| IBIS file bga144.ibs generated by Viper version: 2021.04.12
[IBIS Ver]   5.0
[Comment Char]   |_char
[File Name]   imxrt1180_c0_bga144_consmr.ibs
[File Rev]   1
[Date]   Mon Sep 20 18:29:30 2021
[Source]   NXP Viper 2021.04.12
[Notes]
[Disclaimer] IMPORTANT NOTICE
  This information is provided on an AS IS basis and without warranty.
  IN NO EVENT SHALL NXP BE LIABLE FOR INCIDENTAL OR CONSEQUENTIAL
  DAMAGES ARISING FROM USE OF THIS INFORMATION. THIS DISCLAIMER OF
  WARRANTY EXTENDS TO THE USER OF THE INFORMATION, AND TO THEIR CUSTOMERS
  OR USERS OF PRODUCTS  AND IS IN LIEU OF ALL WARRANTIES WHETHER EXPRESS,
  IMPLIED, OR STATUTORY, INCLUDING IMPLIED WARRANTIES OF MERCHANTABILITY
  OR FITNESS FOR PARTICULAR PURPOSE.
  NXP does not represent or warrant that the information furnished
  hereunder is free of infringement of any third party patents,
  copyrights, trade secrets, or other intellectual property rights.
  NXP does not represent or warrant that the information is free of
  defect, or that it meets any particular standard, requirements or need
  of the user of the infomation or their customers.
  NXP reserves the right to change the information in this file
  without notice.
   http://www.nxp.com
[Copyright]   (C) Copyright NXP 2004 - 2021, All Rights Reserved.
|   BGA144
[Component]   imxrt1180_bga144
[Manufacturer]   NXP
[Package]
| variable   typ   min   max
R_pkg   0.16359   0.065919   0.31382
L_pkg   2.744e-09   1.070e-09   5.893e-09
C_pkg   6.965e-13   4.261e-13   1.190e-12
[Pin] signal_name   model_name   R_pin   L_pin   C_pin
A1   VSS   GND   NA   NA   NA
A2   GPIO_EMC_B1_16   STGPIO   0.28718   5.367e-09 7.642e-13
A3   GPIO_EMC_B1_09   STGPIO   0.22622   3.718e-09 5.945e-13
A4   GPIO_AON_26   FSGPIO   0.16362   2.856e-09 5.265e-13
A5   GPIO_AON_25   FSGPIO   0.17256   2.828e-09 5.105e-13
A6   GPIO_AON_23   FSGPIO   0.19583   3.160e-09 4.965e-13
A7   GPIO_AON_22   FSGPIO   0.18824   3.176e-09 4.828e-13
A8   GPIO_AON_10   FSGPIO   0.16692   2.583e-09 9.013e-13
A9   GPIO_AON_12   FSGPIO   0.24101   4.139e-09 1.094e-12
A10   GPIO_AON_15   FSGPIO   0.3027   5.713e-09 1.030e-12
A11   GPIO_AON_08   FSGPIO   0.31382   5.893e-09 9.051e-13
A12   VSS   GND   NA   NA   NA
B1   GPIO_EMC_B1_15   STGPIO   0.25831   4.469e-09 6.261e-13
B2   GPIO_EMC_B1_11   STGPIO   0.26853   4.818e-09 7.636e-13
B3   GPIO_EMC_B1_17   STGPIO   0.21276   3.476e-09 6.391e-13
B4   GPIO_AON_27   FSGPIO   0.15742   2.693e-09 5.007e-13
B5   GPIO_AON_24   FSGPIO   0.18906   2.825e-09 5.199e-13
B6   GPIO_AON_05   FSGPIO   0.10031   1.570e-09 1.003e-12
B7   GPIO_AON_03   FSGPIO   0.108   2.043e-09 4.957e-13
B8   GPIO_AON_09   FSGPIO   0.16506   2.661e-09 8.544e-13
B9   GPIO_AON_11   FSGPIO   0.23045   3.870e-09 1.087e-12
B10   GPIO_AON_14   FSGPIO   0.29632   5.573e-09 1.094e-12
B11   GPIO_AON_13   FSGPIO   0.30615   5.598e-09 1.046e-12
B12   GPIO_SD_B2_06   STGPIO   0.24063   4.504e-09 6.685e-13
C1   GPIO_EMC_B1_10   STGPIO   0.19712   2.698e-09 4.825e-13
C2   GPIO_EMC_B1_28   STGPIO   0.077242  1.186e-09 7.516e-13
C3   GPIO_EMC_B1_29   STGPIO   0.10015   1.487e-09 6.582e-13
C4   GPIO_AON_17   FSGPIO   0.10536   1.478e-09 6.818e-13
C5   GPIO_AON_16   FSGPIO   0.10709   1.790e-09 6.038e-13
C6   GPIO_AON_02   FSGPIO   0.067407  1.118e-09 1.122e-12
C7   GPIO_AON_01   FSGPIO   0.078667  1.324e-09 1.017e-12
C8   VSS   GND   NA   NA   NA
C9   GPIO_AON_00   FSGPIO   0.19384   3.878e-09 1.009e-12
C10   GPIO_SD_B2_07   STGPIO   0.23187   4.557e-09 7.771e-13
C11   GPIO_SD_B2_11   STGPIO   0.21729   3.877e-09 6.591e-13
C12   GPIO_SD_B2_04   STGPIO   0.19371   3.729e-09 6.738e-13
D1   GPIO_EMC_B1_30   STGPIO   0.18787   2.739e-09 4.927e-13
D2   GPIO_EMC_B1_14   STGPIO   0.11531   2.030e-09 7.770e-13
D3   GPIO_EMC_B1_12   STGPIO   0.067604  1.070e-09 7.102e-13
D4   VSS   GND   NA   NA   NA
D5   NVCC_AON   POWER   NA   NA   NA
D6   GPIO_AON_04   FSGPIO   0.10548   1.871e-09 1.190e-12
D7   GPIO_AON_06   FSGPIO   0.16092   3.123e-09 8.741e-13
D8   GPIO_AON_07   FSGPIO   0.22286   4.219e-09 9.805e-13
D9   VSS   GND   NA   NA   NA
D10   GPIO_SD_B2_05   STGPIO   0.11127   1.889e-09 8.982e-13
D11   GPIO_SD_B2_08   STGPIO   0.16622   2.574e-09 7.092e-13
D12   GPIO_SD_B2_09   STGPIO   0.21685   3.842e-09 5.853e-13
E1   GPIO_EMC_B1_32   STGPIO   0.17445   2.614e-09 4.506e-13
E2   GPIO_EMC_B1_31   STGPIO   0.17592   2.545e-09 4.829e-13
E3   GPIO_EMC_B1_13   STGPIO   0.10229   1.568e-09 8.463e-13
E4   GPIO_AON_21   FSGPIO   0.13406   2.508e-09 8.079e-13
E5   GPIO_AON_20   FSGPIO   0.1388   2.497e-09 8.535e-13
E6   GPIO_AON_19   FSGPIO   0.20153   3.516e-09 9.171e-13
E7   GPIO_AON_18   FSGPIO   0.20448   3.843e-09 9.142e-13
E8   VDD_SOC   POWER   NA   NA   NA
E9   NVCC_SD2   POWER   NA   NA   NA
E10   GPIO_SD_B2_03   STGPIO   0.070294  1.124e-09 8.050e-13
E11   GPIO_SD_B2_01   STGPIO   0.085638  1.305e-09 5.966e-13
E12   GPIO_SD_B2_10   STGPIO   0.16784   2.532e-09 4.453e-13
F1   GPIO_EMC_B1_34   STGPIO   0.17221   2.611e-09 4.420e-13
F2   GPIO_EMC_B1_33   STGPIO   0.18078   2.550e-09 6.132e-13
F3   GPIO_EMC_B1_08   STGPIO   0.11325   1.890e-09 6.770e-13
F4   GPIO_EMC_B1_03   STGPIO   0.11114   2.060e-09 6.860e-13
F5   GPIO_EMC_B1_05   STGPIO   0.11095   2.061e-09 6.978e-13
F6   NVCC_EMC1   POWER   NA   NA   NA
F7   VDD_SOC   POWER   NA   NA   NA
F8   VDD_SOC   POWER   NA   NA   NA
F9   NVCC_SD2   POWER   NA   NA   NA
F10   GPIO_SD_B2_00   STGPIO   0.097558  1.525e-09 6.253e-13
F11   GPIO_SD_B2_02   STGPIO   0.18599   2.795e-09 5.999e-13
F12   ADC_VREFH   NC   0.094419  1.817e-09 5.253e-13
G1   GPIO_EMC_B1_35   STGPIO   0.16837   2.429e-09 4.604e-13
G2   GPIO_EMC_B1_36   STGPIO   0.18715   2.520e-09 6.142e-13
G3   GPIO_EMC_B1_27   STGPIO   0.10364   1.742e-09 6.797e-13
G4   GPIO_EMC_B1_01   STGPIO   0.1415   2.634e-09 7.744e-13
G5   GPIO_EMC_B1_00   STGPIO   0.11834   2.223e-09 7.515e-13
G6   NVCC_EMC1   POWER   NA   NA   NA
G7   VDD_SOC   POWER   NA   NA   NA
G8   VDDA_ADC_3P3   POWER   NA   NA   NA
G9   VDDA_ADC_1P8   POWER   NA   NA   NA
G10   DAC_OUT   NC   0.065919  1.083e-09 6.529e-13
G11   GPIO_AD_30   FSGPIO   0.18141   2.885e-09 5.922e-13
G12   GPIO_AD_31   FSGPIO   0.16864   2.516e-09 4.261e-13
H1   GPIO_EMC_B1_37   STGPIO   0.17602   2.411e-09 5.024e-13
H2   GPIO_EMC_B1_39   STGPIO   0.17575   2.631e-09 4.659e-13
H3   GPIO_EMC_B1_38   STGPIO   0.24055   4.225e-09 7.361e-13
H4   GPIO_EMC_B1_04   STGPIO   0.13736   2.608e-09 7.247e-13
H5   GPIO_EMC_B1_02   STGPIO   0.17915   3.250e-09 7.855e-13
H6   NVCC_EMC1   POWER   NA   NA   NA
H7   GPIO_BBSM_05   NC   0.14691   2.786e-09 8.118e-13
H8   GPIO_BBSM_06   NC   0.13478   2.603e-09 7.785e-13
H9   NVCC_GPIO_AD   POWER   NA   NA   NA
H10   GPIO_AD_18   FSGPIO   0.094077  1.562e-09 6.277e-13
H11   GPIO_AD_19   FSGPIO   0.088023  1.670e-09 4.904e-13
H12   GPIO_AD_29   FSGPIO   0.11929   2.340e-09 4.541e-13
J1   GPIO_EMC_B1_26   STGPIO   0.13411   2.554e-09 4.869e-13
J2   GPIO_EMC_B1_40   STGPIO   0.18514   2.596e-09 5.007e-13
J3   GPIO_EMC_B1_41   STGPIO   0.19787   3.056e-09 5.706e-13
J4   VSS   GND   NA   NA   NA
J5   GPIO_EMC_B1_07   STGPIO   0.12796   2.721e-09 7.157e-13
J6   GPIO_EMC_B1_06   STGPIO   0.1392   3.086e-09 8.299e-13
J7   TEST_MODE   NC   0.25213   4.636e-09 7.670e-13
J8   GPIO_BBSM_00   NC   0.25627   4.609e-09 7.670e-13
J9   VSS   GND   NA   NA   NA
J10   VDDA_1P8_IN   POWER   NA   NA   NA
J11   GPIO_AD_14   FSGPIO   0.10297   1.489e-09 8.353e-13
J12   GPIO_AD_15   FSGPIO   0.10216   1.657e-09 6.078e-13
K1   DCDC_SENSE   POWER   0.18582   2.383e-09 4.766e-13
K2   DCDC_PSWITCH   NC   0.18656   2.611e-09 4.898e-13
K3   DCDC_GND   GND   NA   NA   NA
K4   DCDC_IN_Q   POWER   0.088509  1.651e-09 7.551e-13
K5   ONOFF   NC   0.20344   3.359e-09 6.540e-13
K6   GPIO_BBSM_01   NC   0.073539  1.216e-09 6.201e-13
K7   NVCC_BBSM   POWER   NA   NA   NA
K8   VDD_BBSM_ANA   POWER   NA   NA   NA
K9   VDD_AON_ANA   POWER   NA   NA   NA
K10   GPIO_AD_13   FSGPIO   0.085008  1.325e-09 7.009e-13
K11   GPIO_AD_12   FSGPIO   0.22058   3.187e-09 8.131e-13
K12   GPIO_AD_17   FSGPIO   0.22522   3.387e-09 6.835e-13
L1   DCDC_1P8   POWER   0.086379  1.798e-09 7.307e-13
L2   DCDC_LP   POWER   NA   NA   NA
L3   DCDC_GND   GND   NA   NA   NA
L4   DCDC_IN   POWER   NA   NA   NA
L5   PMIC_ON_REQ   NC   0.17119   2.572e-09 5.895e-13
L6   POR_B   NC   0.16787   2.505e-09 5.617e-13
L7   RTC_XTALO   NC   0.10473   1.522e-09 5.551e-13
L8   VDD_AON_IN   POWER   NA   NA   NA
L9   XTALO   NC   0.11074   1.571e-09 5.999e-13
L10   VSS   GND   NA   NA   NA
L11   CLK1_N   NC   0.21895   3.146e-09 7.817e-13
L12   GPIO_AD_16   FSGPIO   0.22382   3.398e-09 7.083e-13
M1   VSS   GND   NA   NA   NA
M2   DCDC_LP   POWER   NA   NA   NA
M3   DCDC_GND   GND   NA   NA   NA
M4   DCDC_IN   POWER   NA   NA   NA
M5   WAKEUP   NC   0.178   2.735e-09 5.291e-13
M6   VDD_BBSM_IN   POWER   NA   NA   NA
M7   RTC_XTALI   NC   0.11374   1.747e-09 5.677e-13
M8   VDD_AON_DIG   POWER   NA   NA   NA
M9   XTALI   NC   0.11181   1.555e-09 6.216e-13
M10   VDDA_1P0   POWER   NA   NA   NA
M11   CLK1_P   NC   0.22364   3.329e-09 7.427e-13
M12   VSS   GND   NA   NA   NA
[Pin Mapping]   pulldown_ref   pullup_ref
A1   VSS   NC
A2   VSS   NVCC_EMC1
A3   VSS   NVCC_EMC1
A4   VSS   NVCC_AON
A5   VSS   NVCC_AON
A6   VSS   NVCC_AON
A7   VSS   NVCC_AON
A8   VSS   NVCC_AON
A9   VSS   NVCC_AON
A10   VSS   NVCC_AON
A11   VSS   NVCC_AON
A12   VSS   NC
B1   VSS   NVCC_EMC1
B2   VSS   NVCC_EMC1
B3   VSS   NVCC_EMC1
B4   VSS   NVCC_AON
B5   VSS   NVCC_AON
B6   VSS   NVCC_AON
B7   VSS   NVCC_AON
B8   VSS   NVCC_AON
B9   VSS   NVCC_AON
B10   VSS   NVCC_AON
B11   VSS   NVCC_AON
B12   VSS   NVCC_SD2
C1   VSS   NVCC_EMC1
C2   VSS   NVCC_EMC1
C3   VSS   NVCC_EMC1
C4   VSS   NVCC_AON
C5   VSS   NVCC_AON
C6   VSS   NVCC_AON
C7   VSS   NVCC_AON
C8   VSS   NC
C9   VSS   NVCC_AON
C10   VSS   NVCC_SD2
C11   VSS   NVCC_SD2
C12   VSS   NVCC_SD2
D1   VSS   NVCC_EMC1
D2   VSS   NVCC_EMC1
D3   VSS   NVCC_EMC1
D4   VSS   NC
D5   NC   NVCC_AON
D6   VSS   NVCC_AON
D7   VSS   NVCC_AON
D8   VSS   NVCC_AON
D9   VSS   NC
D10   VSS   NVCC_SD2
D11   VSS   NVCC_SD2
D12   VSS   NVCC_SD2
E1   VSS   NVCC_EMC1
E2   VSS   NVCC_EMC1
E3   VSS   NVCC_EMC1
E4   VSS   NVCC_AON
E5   VSS   NVCC_AON
E6   VSS   NVCC_AON
E7   VSS   NVCC_AON
E8   NC   VDD_SOC
E9   NC   NVCC_SD2
E10   VSS   NVCC_SD2
E11   VSS   NVCC_SD2
E12   VSS   NVCC_SD2
F1   VSS   NVCC_EMC1
F2   VSS   NVCC_EMC1
F3   VSS   NVCC_EMC1
F4   VSS   NVCC_EMC1
F5   VSS   NVCC_EMC1
F6   NC   NVCC_EMC1
F7   NC   VDD_SOC
F8   NC   VDD_SOC
F9   NC   NVCC_SD2
F10   VSS   NVCC_SD2
F11   VSS   NVCC_SD2
F12   NC   NC
G1   VSS   NVCC_EMC1
G2   VSS   NVCC_EMC1
G3   VSS   NVCC_EMC1
G4   VSS   NVCC_EMC1
G5   VSS   NVCC_EMC1
G6   NC   NVCC_EMC1
G7   NC   VDD_SOC
G8   NC   VDDA_ADC_3P3
G9   NC   VDDA_ADC_1P8
G10   NC   NC
G11   VSS   NVCC_GPIO_AD
G12   VSS   NVCC_GPIO_AD
H1   VSS   NVCC_EMC1
H2   VSS   NVCC_EMC1
H3   VSS   NVCC_EMC1
H4   VSS   NVCC_EMC1
H5   VSS   NVCC_EMC1
H6   NC   NVCC_EMC1
H7   NC   NC
H8   NC   NC
H9   NC   NVCC_GPIO_AD
H10   VSS   NVCC_GPIO_AD
H11   VSS   NVCC_GPIO_AD
H12   VSS   NVCC_GPIO_AD
J1   VSS   NVCC_EMC1
J2   VSS   NVCC_EMC1
J3   VSS   NVCC_EMC1
J4   VSS   NC
J5   VSS   NVCC_EMC1
J6   VSS   NVCC_EMC1
J7   NC   NC
J8   NC   NC
J9   VSS   NC
J10   NC   VDDA_1P8_IN
J11   VSS   NVCC_GPIO_AD
J12   VSS   NVCC_GPIO_AD
K1   NC   DCDC_SENSE
K2   NC   NC
K3   DCDC_GND   NC
K4   NC   DCDC_IN_Q
K5   NC   NC
K6   NC   NC
K7   NC   NVCC_BBSM
K8   NC   VDD_BBSM_ANA
K9   NC   VDD_AON_ANA
K10   VSS   NVCC_GPIO_AD
K11   VSS   NVCC_GPIO_AD
K12   VSS   NVCC_GPIO_AD
L1   NC   DCDC_1P8
L2   NC   DCDC_LP
L3   DCDC_GND   NC
L4   NC   DCDC_IN
L5   NC   NC
L6   NC   NC
L7   NC   NC
L8   NC   VDD_AON_IN
L9   NC   NC
L10   VSS   NC
L11   NC   NC
L12   VSS   NVCC_GPIO_AD
M1   VSS   NC
M2   NC   DCDC_LP
M3   DCDC_GND   NC
M4   NC   DCDC_IN
M5   NC   NC
M6   NC   VDD_BBSM_IN
M7   NC   NC
M8   NC   VDD_AON_DIG
M9   NC   NC
M10   NC   VDDA_1P0
M11   NC   NC
M12   VSS   NC
|*   Model Selector   *
[Model Selector] STGPIO
BDPROGSCARUDQP_SDMMC_3V3SF_00_SD   PSW=0 High Drive, 1V8 SD
BDPROGSCARUDQP_SDMMC_3V3SF_01_SD   PSW=0 Low Drive,  1V8 SD
BDPROGSCARUDQP_SDMMC_3V3SF_00_MMC   PSW=0 High Drive, 1V8 MMC
BDPROGSCARUDQP_SDMMC_3V3SF_01_MMC   PSW=0 Low Drive,  1V8 MMC
BDPROGSCARUDQP_SDMMC_3V3SF_10   PSW=1 High Drive, 3V3 +/- 10%, SD & 3V3 MMC
BDPROGSCARUDQP_SDMMC_3V3SF_11   PSW=1 Low Drive,  3V3 +/- 10%, SD & 3V3 MMC
BDPROGSCARUDQP_SDMMC_3V3SF_10_5pct  PSW=1 High Drive, 3V3 +/- 5%, SD & 3V3 MMC
BDPROGSCARUDQP_SDMMC_3V3SF_11_5pct  PSW=1 Low Drive,  3V3 +/- 5%, SD & 3V3 MMC
BDPROGSCARUDQP_SDMMC_3V3SF_11_2v7   PSW=1 Low Drive,  2V7 SD & 2V7 MMC
BDPROGSCARUDQP_SDMMC_3V3SF_10_2v7   PSW=1 High Drive, 2V7 SD & 2V7 MMC
[Model Selector] FSGPIO
io_crnrobe1dse0sre0   Normal range in cont mode, 5mA drive strength, without slew rate
io_crnrobe1dse0sre1   Normal range in cont mode, 5mA drive strength, with slew rate
io_crnrobe1dse1sre0   Normal range in cont mode, 10mA drive strength, without slew rate
io_crnrobe1dse1sre1   Normal range in cont mode, 10mA drive strength, with slew rate
io_crdrobe1dse0sre0   Derated range in cont mode, 5mA drive strength, without slew rate
io_crdrobe1dse0sre1   Derated range in cont mode, 5mA drive strength, with slew rate
io_crdrobe1dse1sre0   Derated range in cont mode, 10mA drive strength, without slew rate
io_crdrobe1dse1sre1   Derated range in cont mode, 10mA drive strength, with slew rate
io_crdr2obe1dse0sre0   Derated2 range in cont mode, 5mA drive strength, without slew rate
io_crdr2obe1dse0sre1   Derated2 range in cont mode, 5mA drive strength, with slew rate
io_crdr2obe1dse1sre0   Derated2 range in cont mode, 10mA drive strength, without slew rate
io_crdr2obe1dse1sre1   Derated2 range in cont mode, 10mA drive strength, with slew rate
io_hrobe1dse0sre0   high range mode, 5mA drive strength, without slew rate
io_hrobe1dse0sre1   high range mode, 5mA drive strength, with slew rate
io_hrobe1dse1sre0   high range mode, 10mA drive strength, without slew rate
io_hrobe1dse1sre1   high range mode, 10mA drive strength, with slew rate
io_lrobe1dse0sre0   low range mode, 5mA drive strength, without slew rate
io_lrobe1dse0sre1   low range mode, 5mA drive strength, with slew rate
io_lrobe1dse1sre0   low range mode, 10mA drive strength, without slew rate
io_lrobe1dse1sre1   low range mode, 10mA drive strength, with slew rate
io_crnrobe1dse0sre0_5pct   Narrow range in cont mode, 5mA drive strength, without slew rate
io_crnrobe1dse0sre1_5pct   Narrow range in cont mode, 5mA drive strength, with slew rate
io_crnrobe1dse1sre0_5pct   Narrow range in cont mode, 10mA drive strength, without slew rate
io_crnrobe1dse1sre1_5pct   Narrow range in cont mode, 10mA drive strength, with slew rate
io_hrobe1dse0sre0_5pct   Narrow range in high range mode, 5mA drive strength, without slew rate
io_hrobe1dse0sre1_5pct   Narrow range in high range mode, 5mA drive strength, with slew rate
io_hrobe1dse1sre0_5pct   Narrow range in high range mode, 10mA drive strength, without slew rate
io_hrobe1dse1sre1_5pct   Narrow range in high range mode, 10mA drive strength, with slew rate
|End  [Component] imxrt1180_bga144
| Models and submodels in the file (38): BDPROGSCARUDQP_SDMMC_3V3SF_00_MMC (I/O), BDPROGSCARUDQP_SDMMC_3V3SF_00_SD (I/O), BDPROGSCARUDQP_SDMMC_3V3SF_01_MMC (I/O), BDPROGSCARUDQP_SDMMC_3V3SF_01_SD (I/O), BDPROGSCARUDQP_SDMMC_3V3SF_10 (I/O), BDPROGSCARUDQP_SDMMC_3V3SF_11 (I/O), BDPROGSCARUDQP_SDMMC_3V3SF_10_2v7 (I/O), BDPROGSCARUDQP_SDMMC_3V3SF_11_2v7 (I/O), BDPROGSCARUDQP_SDMMC_3V3SF_10_5pct (I/O), BDPROGSCARUDQP_SDMMC_3V3SF_11_5pct (I/O), io_crnrobe1dse0sre0 (I/O), io_crnrobe1dse0sre1 (I/O), io_crnrobe1dse1sre0 (I/O), io_crnrobe1dse1sre1 (I/O), io_crdrobe1dse0sre0 (I/O), io_crdrobe1dse0sre1 (I/O), io_crdrobe1dse1sre0 (I/O), io_crdrobe1dse1sre1 (I/O), io_crdr2obe1dse0sre0 (I/O), io_crdr2obe1dse0sre1 (I/O), io_crdr2obe1dse1sre0 (I/O), io_crdr2obe1dse1sre1 (I/O), io_hrobe1dse0sre0 (I/O), io_hrobe1dse0sre1 (I/O), io_hrobe1dse1sre0 (I/O), io_hrobe1dse1sre1 (I/O), io_lrobe1dse0sre0 (I/O), io_lrobe1dse0sre1 (I/O), io_lrobe1dse1sre0 (I/O), io_lrobe1dse1sre1 (I/O), io_crnrobe1dse0sre0_5pct (I/O), io_crnrobe1dse0sre1_5pct (I/O), io_crnrobe1dse1sre0_5pct (I/O), io_crnrobe1dse1sre1_5pct (I/O), io_hrobe1dse0sre0_5pct (I/O), io_hrobe1dse0sre1_5pct (I/O), io_hrobe1dse1sre0_5pct (I/O), io_hrobe1dse1sre1_5pct (I/O)
